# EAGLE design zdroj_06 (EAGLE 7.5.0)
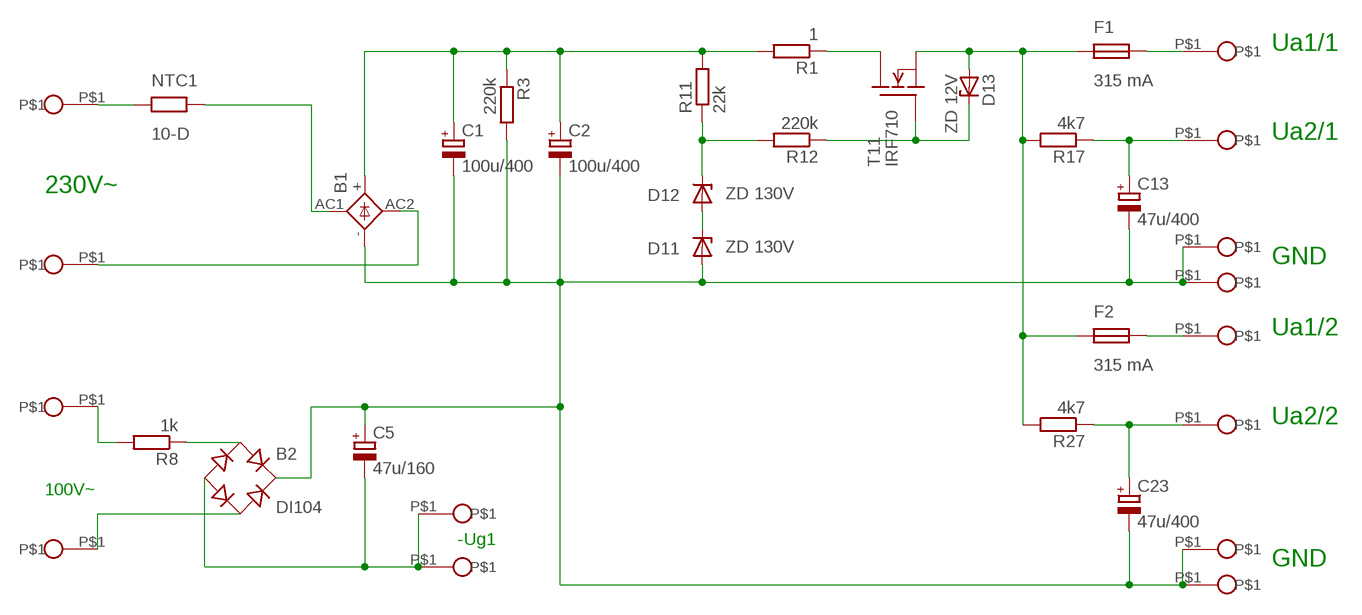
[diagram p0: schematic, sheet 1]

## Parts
B1  FB15  [FB15]
B2  DI104  B-DIL  [B-DIL]
C1  100u/400  CPOL-EUE7.5-18  [E7,5-18]
C2  100u/400  CPOL-EUE7.5-18  [E7,5-18]
C5  47u/160  CPOL-EUE5-10.5  [E5-10,5]
C13  47u/400  CPOL-EUE7.5-16  [E7,5-16]
C23  47u/400  CPOL-EUE7.5-16  [E7,5-16]
D11  ZD 130V  BZW03XX  [SOD64Z12]
D12  ZD 130V  BZW03XX  [SOD64Z12]
D13  ZD 12V  BZW03XX  [SOD64Z12]
F1  315 mA  FUSEF1  [FUSE]
F2  315 mA  FUSEF1  [FUSE]
NTC1  10-D  R2W  [R2W]
R1  1  R-EU_0207/10  [0207/10]
R3  220k  R-EU_0207/10  [0207/10]
R8  1k  R-EU_0207/10  [0207/10]
R11  22k  R-EU_0207/10  [0207/10]
R12  220k  R-EU_0207/10  [0207/10]
R17  4k7  R-EU_0207/10  [0207/10]
R27  4k7  R-EU_0207/10  [0207/10]
T11  IRF710  IRF840V  [TO220V]
U$2  PIN  [PIN]
U$3  PIN  [PIN]
U$4  PIN  [PIN]
U$5  PIN  [PIN]
U$7  PIN  [PIN]
U$8  PIN  [PIN]
U$11  PIN  [PIN]
U$15  PIN  [PIN]
U$16  PIN  [PIN]
U$17  PIN  [PIN]
U$18  PIN  [PIN]
U$20  PIN  [PIN]
U$26  PIN  [PIN]
U$29  PIN  [PIN]

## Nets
GND: B1.- B2.+ C1.- C2.- C5.+ C13.- C23.- D11.A R3.2 U$2.P$1 U$7.P$1 U$8.P$1 U$29.P$1
GND2: B2.- C5.- U$18.P$1 U$26.P$1
N$1: D13.A F1.P$2 F2.P$2 R17.2 R27.2 T11.3(S)
N$2: R1.1 T11.2(D)
N$3: D11.C D12.A
N$4: D12.C R11.1 R12.2
N$5: B1.+ C1.+ C2.+ R1.2 R3.1 R11.2
N$6: B2.AC1 R8.1
N$7: F1.P$4 U$20.P$1
N$8: F2.P$4 U$4.P$1
N$9: B1.AC1 NTC1.2
N$10: B1.AC2 U$11.P$1
N$15: NTC1.1 U$5.P$1
N$18: B2.AC2 U$17.P$1
N$21: C13.+ R17.1 U$16.P$1
N$22: C23.+ R27.1 U$3.P$1
N$28: R8.2 U$15.P$1
N$35: D13.C R12.1 T11.1(G)

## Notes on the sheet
- Ua1/1
- Ua2/1
- 230V~
- GND
- Ua1/2
- Ua2/2
- 100V~
- -Ug1
- GND

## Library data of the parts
B1 = rectifier:FB15: FAGOR RECTIFIER grid 3 x 5 mm
B2 = rectifier:B-DIL: RECTIFIER
C1 C2 C5 C13 C23 = rcl:CPOL-EU: POLARIZED CAPACITOR, European symbol
D11-D13 = diode:BZW03XX: Z DIODE
F1 F2 = lampy03:FUSE
NTC1 = LAMPY02:R2W
R1 R3 R8 R11 R12 R17 R27 = rcl:R-EU_: RESISTOR, European symbol
T11 = transistor-fet:IRF840: N-Channel Enhancement MOSFET (HEXFET); 500V; 8A; 0,85Ohm
U$2-U$5 U$7 U$8 U$11 U$15-U$18 U$20 U$26 U$29 = LAMPY02:PIN

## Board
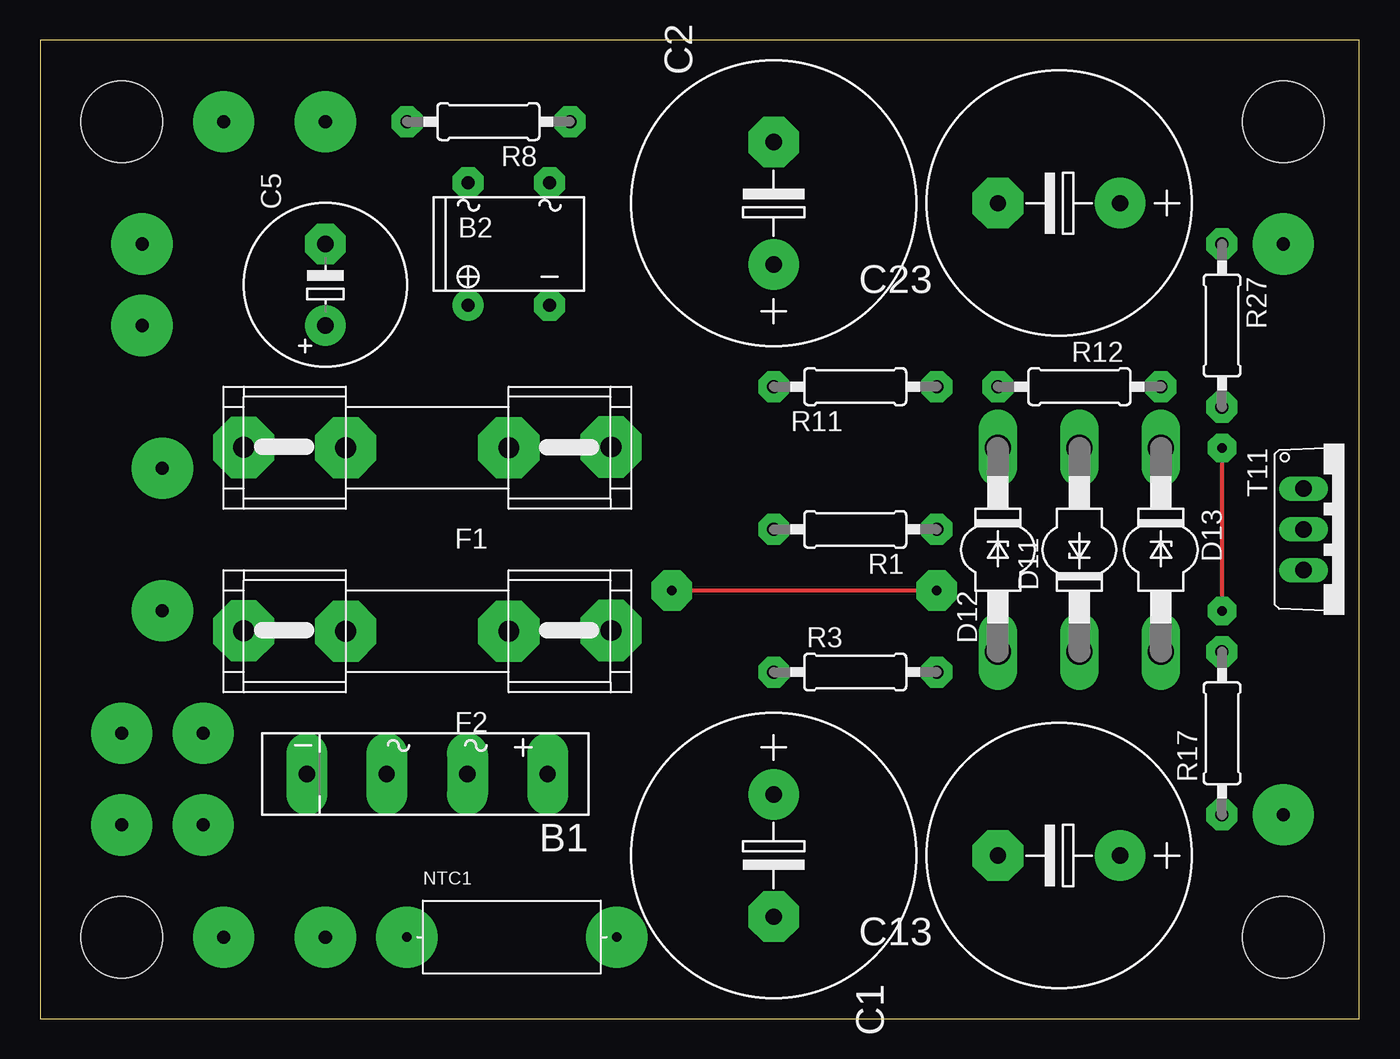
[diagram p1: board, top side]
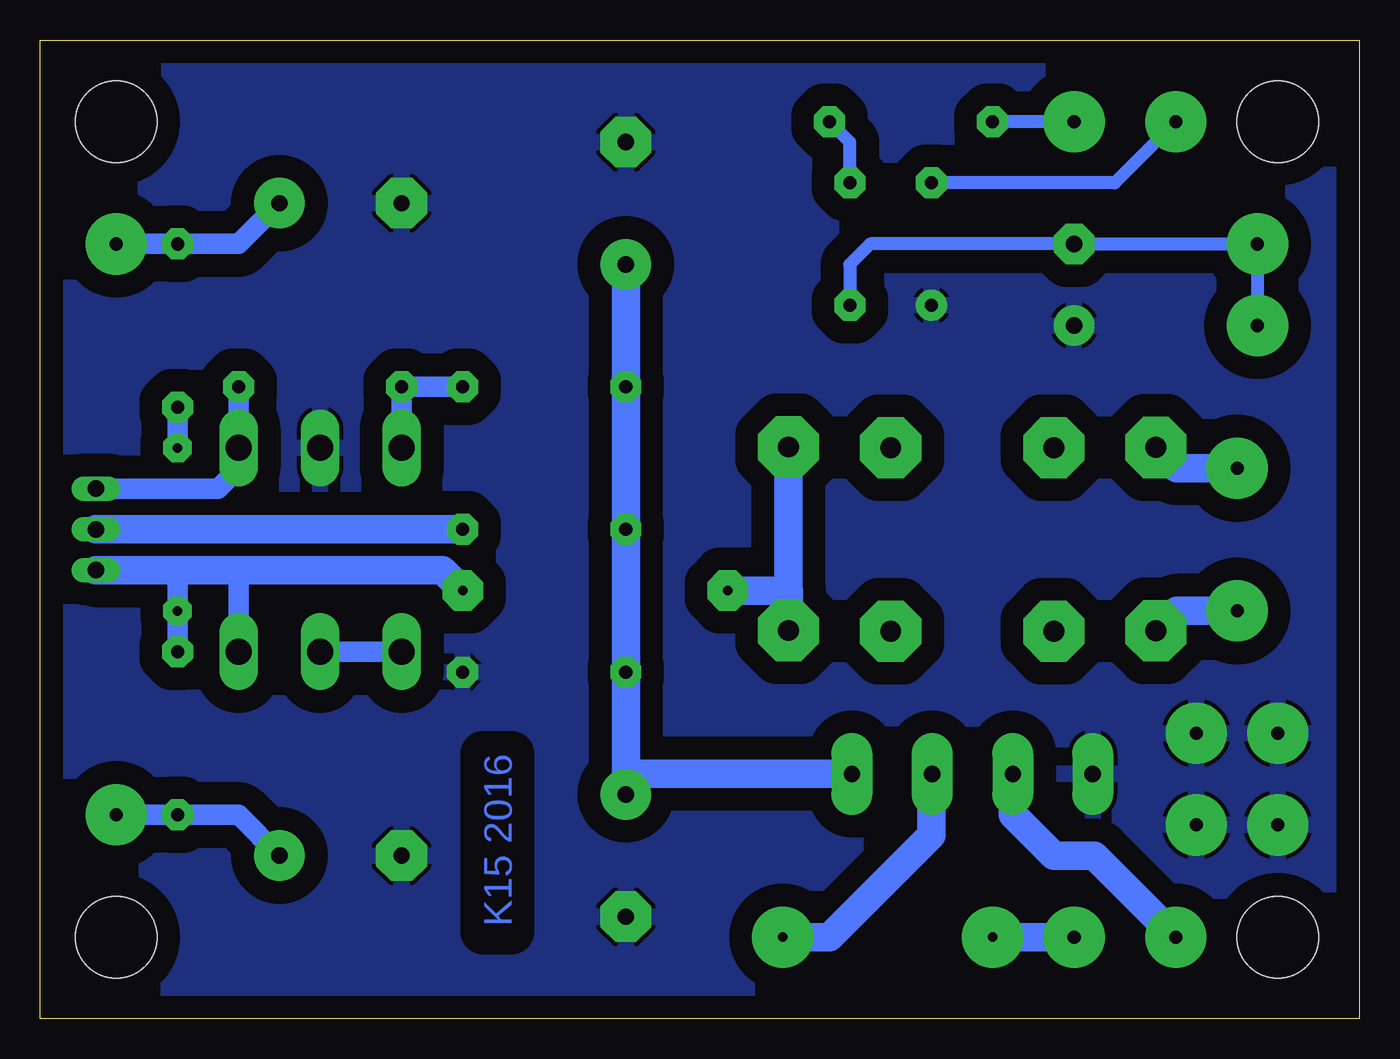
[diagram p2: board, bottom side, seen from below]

Size 82.22 x 60.96 mm. Coordinates in mm from the lower left corner, seen from the top.
Outline: 0,0 82.22,0 82.22,60.95 78.74,60.96 0,60.96 0,0
Copper layers (1*16): Top 0.035mm / dielectric 1.5mm / Bottom 0.035mm
Design rules "default": minimum track width 10mil, minimum drill 24mil, track to track 8mil, track to pad 8mil, pad to pad 8mil, via to via 8mil, smd to smd 8mil, copper to edge 40mil, drill to drill 8mil, minimum pad ring 10mil, minimum via ring 8mil, stop-mask expansion 4mil, vias tented up to drill 0mil, thermal gap 10mil
Holes 5.08 mm at 77.47,55.88 77.47,5.08 5.08,55.88 5.08,5.08

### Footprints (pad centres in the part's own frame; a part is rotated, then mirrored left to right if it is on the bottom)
FB15 = drill 1.016 pad 2.54 long: + -7.5,0; - 7.511,0; AC1 -2.496,0; AC2 2.533,0
B-DIL = drill 0.813 pad 1.93: + -2.54,-3.81 | drill 0.813 pad 1.93 octagon: - 2.54,-3.81; AC1 2.54,3.81; AC2 -2.54,3.81
E7,5-18 = drill 1.016 pad 3.15: + -3.81,0 | drill 1.016 pad 3.15 octagon: - 3.81,0
E5-10,5 = drill 1.016 pad 2.54: + -2.54,0 | drill 1.016 pad 2.54 octagon: - 2.54,0
E7,5-16 = drill 1.016 pad 3.15: + -3.81,0 | drill 1.016 pad 3.15 octagon: - 3.81,0
SOD64Z12 = drill 1.6 long: A 6.35,0; C -6.35,0
FUSE = drill 1.3 pad 3.81 octagon: P$1 -5.08,0; P$2 -11.448,-0.051; P$3 5.08,0; P$4 11.448,-0.025
R2W = drill 0.61 pad 3.81: 1 0,0; 2 13.08,0
0207/10 = drill 0.813 pad 1.93 octagon: 1 -5.08,0; 2 5.08,0
TO220V = drill 1.016 long: 1 -2.54,-2.54; 2 0,-2.54; 3 2.54,-2.54
PIN = drill 0.813 pad 3.81: P$1 0,0

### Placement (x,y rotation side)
B1  24.13,15.24 180 top
B2  29.21,48.26 0 top
C1  45.72,10.16 270 top
C2  45.72,50.8 90 top
C5  17.78,45.72 90 top
C13  63.5,10.16 180 top
C23  63.5,50.8 180 top
D11  64.77,29.21 90 top
D12  59.69,29.21 270 top
D13  69.85,29.21 270 top
F1  24.13,35.56 180 top
F2  24.13,24.13 180 top
NTC1  22.86,5.08 0 top
R1  50.8,30.48 180 top
R3  50.8,21.59 0 top
R8  27.94,55.88 180 top
R11  50.8,39.37 180 top
R12  64.77,39.37 180 top
R17  73.66,17.78 90 top
R27  73.66,43.18 270 top
T11  81.28,30.48 270 top
U$2  5.08,17.78 0 top
U$3  77.47,48.26 0 top
U$4  7.62,25.4 0 top
U$5  17.78,5.08 0 top
U$7  10.16,12.06 0 top
U$8  5.08,12.06 0 top
U$11  11.43,5.08 0 top
U$15  17.78,55.88 0 top
U$16  77.47,12.7 0 top
U$17  11.43,55.88 0 top
U$18  6.35,48.26 0 top
U$20  7.62,34.29 0 top
U$26  6.35,43.18 0 top
U$29  10.16,17.78 0 top

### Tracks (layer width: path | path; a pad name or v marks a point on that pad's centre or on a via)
GND
  pour Bottom (isolate 1.422): 0,62.23 82.55,62.23 82.55,0 0,0
GND2
  Bottom 0.813: U$26.P$1 U$18.P$1 C5.- 30.48,48.26 31.75,46.99 B2.-
N$1  (via drill 0.6 pad 1.78, 0.6 pad 2.54)
  Top 0.254: v55.88,26.67 v39.37,26.67 | v73.66,35.56 v73.66,25.4
  Bottom 1.27: D13.A 69.85,27.94 | R17.2 v73.66,25.4 73.66,27.94 | R27.2 v73.66,35.56
  Bottom 1.778: T11.3 73.66,27.94 69.85,27.94 57.15,27.94 v55.88,26.67 | v39.37,26.67 35.56,26.67 35.56,26.07 | 35.56,25.4 35.56,26.07 | 35.56,26.07 F2.P$2 F1.P$2
N$2
  Bottom 1.778: R1.1 T11.2
N$3
  Bottom 1.27: D12.A D11.C
N$4
  Bottom 1.27: R11.1 R12.2 D12.C
N$5
  Bottom 1.778: B1.+ 45.72,15.24 | C1.+ 45.72,15.24 | 45.72,15.24 R3.1 R1.2 R11.2 C2.+
N$6
  Bottom 0.813: B2.AC1 31.75,54.61 R8.1
N$7
  Bottom 1.778: U$20.P$1 11.39,34.29 F1.P$4
N$8
  Bottom 1.778: U$4.P$1 11.39,25.4 F2.P$4
N$9
  Bottom 1.778: NTC1.2 33.02,5.08 26.67,11.43 26.67,15.2 B1.AC1
N$10
  Bottom 1.778: U$11.P$1 16.51,10.16 19.05,10.16 21.59,12.7 B1.AC2
N$15
  Bottom 1.778: U$5.P$1 NTC1.1
N$18
  Bottom 0.813: U$17.P$1 15.24,52.07 B2.AC2
N$21
  Bottom 1.27: U$16.P$1 R17.1 69.85,12.7 C13.+
N$22
  Bottom 1.27: U$3.P$1 R27.1 69.85,48.26 C23.+
N$28
  Bottom 0.813: U$15.P$1 R8.2
N$35
  Bottom 1.27: T11.1 71.12,33.02 69.85,34.29 D13.C R12.1

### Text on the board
Bottom: K15 2016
